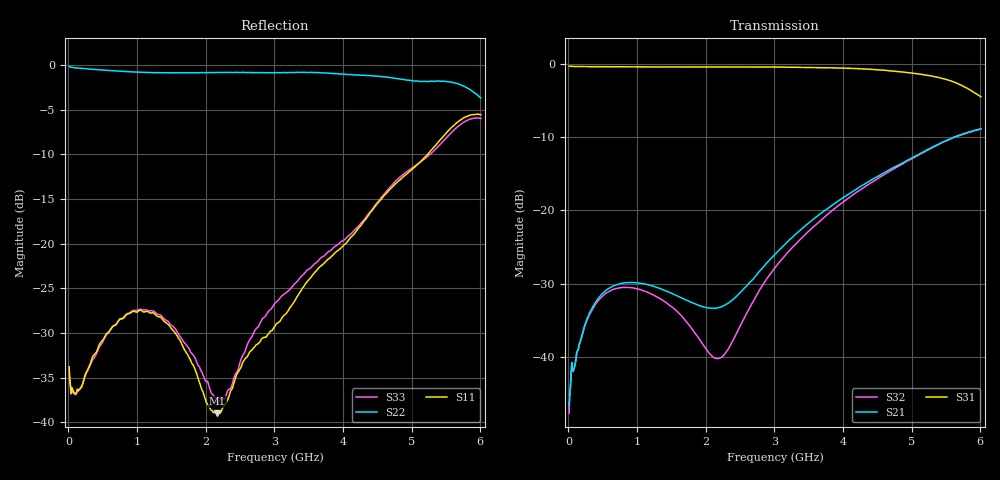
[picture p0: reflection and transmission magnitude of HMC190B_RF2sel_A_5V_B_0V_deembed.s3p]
! Device:	HMC190B
! Description:	GaAs MMIC SPDT Reflective Switch
! Package:	8-lead mini small outline package
! Frequency:	DC -  3 GHz
! Ports:
! RFC = Port 1
! RF1 = Port 2
! RF2 = Port 3
! State: RF2 Selected
! Control Voltages:
! A  = 5 V
! B  = 0 V
! Data:	Data was collected using a calibrated network analyzer with AFR software.
!	Fixtures were calculated using AFR and fixturing was applied to collect
!	this Deembedded  S Parameter data of HMC190B.
! Note:	Analog Devices supplies this data as a sample of measured data at the package pin
!	for this product.  Your particular data for this product may vary.
!	Data was taken at 25 degrees C.
!	Analog Devices reserves the right to change this data at anytime.
# Hz S  dB  R 50
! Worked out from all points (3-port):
!   601 points, 10 MHz to 6.01 GHz, reference 50 ohm
!   strongest paths, dB at 10 MHz, 1.51 GHz, 3.01 GHz, 4.51 GHz, 6.01 GHz:
!     S31: -0.3, -0.4, -0.4, -0.8, -4.5
!     S21: -46.8, -31.4, -26.0, -15.3, -8.8
!     S32: -47.7, -33.2, -27.8, -15.6, -8.9
!   lowest |S11| = -39.0 dB at 2.17 GHz (marker M1), VSWR 1.02, Z = 49.2 + j0.751 ohm
!   |S11| at or under -10 dB: start of sweep to 5.236 GHz
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1e7  -33.77 -6.5  -46.92 12.5  -0.28 -0.4
     -46.80 16.0  -0.15 -2.8  -47.49 14.3
     -0.28 -0.5  -47.72 16.7  -34.65 -6.8
2.7e8  -34.27 44.3  -34.80 47.8  -0.34 -5.6
       -34.82 47.6  -0.44 -54.7  -35.02 40.2
       -0.34 -5.6  -35.02 40.3  -34.35 37.6
5.1e8  -30.70 56.8  -31.23 38.7  -0.36 -10.5
       -31.24 38.6  -0.59 -93.2  -31.63 25.4
       -0.36 -10.5  -31.61 25.3  -30.80 51.4
7.9e8  -28.37 61.1  -29.93 28.0  -0.37 -16.2
       -29.94 28.0  -0.73 -125.8  -30.53 6.7
       -0.37 -16.2  -30.53 6.7  -28.34 52.0
1.13e9  -27.59 64.3  -30.07 20.5  -0.38 -23.1
        -30.08 20.5  -0.85 -153.5  -31.09 -12.7
        -0.38 -23.0  -31.09 -12.7  -27.41 42.3
2.17e9  -38.97 137.3  -33.32 50.2  -0.38 -44.5
        -33.31 50.2  -0.85 158.4  -40.23 -116.6
        -0.38 -44.5  -40.25 -116.6  -37.77 -44.9
3.01e9  -29.23 -167.5  -25.99 85.7  -0.40 -62.7
        -26.00 85.7  -0.88 129.5  -27.82 137.5
        -0.40 -62.7  -27.82 137.5  -26.66 -127.5
4.55e9  -15.11 146.1  -15.11 60.8  -0.80 -100.7
        -15.11 60.9  -1.31 81.3  -15.37 75.3
        -0.80 -100.7  -15.38 75.3  -14.92 -175.6
5.38e9  -8.71 123.0  -11.01 38.7  -1.80 -124.9
        -11.02 38.7  -1.80 64.4  -11.07 45.3
        -1.79 -124.9  -11.07 45.3  -9.19 148.7
6.01e9  -5.57 117.2  -8.84 19.3  -4.46 -142.5
        -8.84 19.3  -3.71 61.0  -8.86 20.9
        -4.46 -142.5  -8.86 20.9  -5.99 127.7
